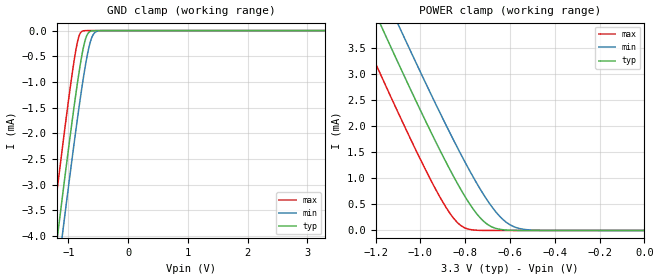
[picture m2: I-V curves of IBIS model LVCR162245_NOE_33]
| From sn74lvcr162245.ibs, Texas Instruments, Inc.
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[Model]   LVCR162245_NOE_33
Model_type  Input
Vinl=0.8
Vinh=2.0
| variable   typ   min   max
C_comp   1.22pF   1.04pF   2.05pF
[Temperature Range]   40   100   -40
| Ambient temperature   25   85   -40
[Voltage range]   3.3   3   3.6
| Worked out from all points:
|   GND clamp passes 1 mA (typ) near -0.85 V on its own axis
|   POWER clamp passes 1 mA (typ) near -0.85 V on its own axis
[GND Clamp]
| LVCR162245_NOE_33
|   Voltage   I(typ)   I(min)   I(max)
-5.5V     -46.83mA   -47.49mA   -46mA
-1.29V    -5.015mA   -5.753mA   -4.062mA
-1.255V   -4.681mA   -5.42mA    -3.727mA
-1.19V    -4.065mA   -4.805mA   -3.109mA
-1.16V    -3.783mA   -4.522mA   -2.827mA
-1.105V   -3.269mA   -4.008mA   -2.314mA
-930mV    -1.689mA   -2.412mA   -776uA
-835mV    -905.1uA   -1.593mA   -153.9uA
-705mV    -131.6uA   -603.9uA   -580.2nA
-625mV    -11.21uA   -186.8uA   -11.91nA
-550mV    -770.8nA   -30.65uA   -319.3pA
3.3V      6.303pA    16.94nA    5.63pA
[POWER Clamp]
| LVCR162245_NOE_33
|   Voltage   I(typ)   I(min)   I(max)
-5.5V     46.83mA    47.49mA    46mA
-1.325V   5.35mA     6.087mA    4.398mA
-1.26V    4.729mA    5.468mA    3.775mA
-1.155V   3.736mA    4.476mA    2.78mA
-1.085V   3.084mA    3.822mA    2.129mA
-935mV    1.732mA    2.457mA    816uA
-840mV    943.8uA    1.634mA    176.2uA
-795mV    611.2uA    1.266mA    38.41uA
-725mV    207uA      738.7uA    1.527uA
-620mV    9.413uA    169.2uA    9.346nA
-500mV    126.5nA    7.204uA    35.76pA
-95.1fV   6.303pA    7.801pA    6.677pA
